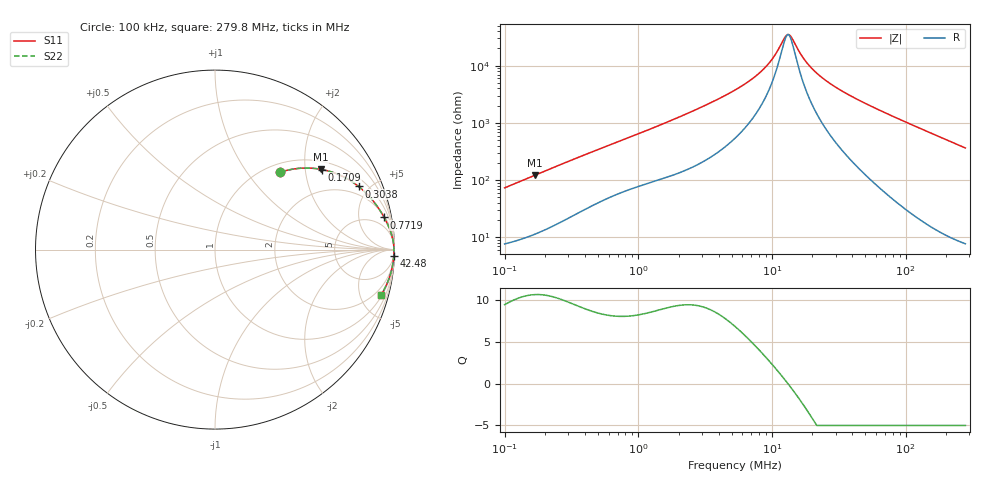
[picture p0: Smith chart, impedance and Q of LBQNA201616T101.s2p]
! LBQNA201616T101  S-PARAMETER MODEL  ( General Type )
! Model Generated by TAIYO YUDEN Corporation (http://www.ty-top.com)
! Version 1.0
! TAIYO YUDEN Control No. 191025NI43SB-FBB
! Copyright(c) 2019 TAIYO YUDEN CO.,LTD. All Rights Reserved.
! Product Description (link to TY-COMPAS)
! https://ds.yuden.co.jp/TYCOMPAS/or/detail?pn=LBQNA201616T101K&u=M
! Products Name : Inductors
! Characteristics :
!  Inductance : 100 uH , SRF(min) : 8.0 MHz , DC Resistance(max) : 5.85 Ohm
!  Rated Current : Saturation :70 mA , Temp Rise : 90 mA (20 degC)
!  Case Size : 2.0 x 1.6 / 0.079 x 0.063 [mm/inch] , Thickness : 1.6 / 0.063 [mm/inch]
!  (Conditions: Temperature = 25 degC , DC Bias Current/Voltage = 0A / 0V)
! External Node Assignments :
!  1  o---GGG---o  2
! GND o---------o GND
! Frequency Range : 0.1MHz  -  279.750408MHz  [ 402 STEP ]
# MHz S RI R 50
! Freq[MHz].  S11 Real  S11 Imag  S21 Real  S21 Imag  S12 Real  S12 Imag  S22 Real  S22 Imag
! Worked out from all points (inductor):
!   401 points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, 100 kHz to 279.8 MHz, reference 50 ohm
!   read as one part in series: L = 116 uH near 104 kHz
!   highest Q = 10.7 at 167.5 kHz (marker M1), where L = 115 uH
!   self-resonance near 13.18 MHz
!   S11 on the Smith chart (normalised r, x): 100 kHz: 1.15, +1.46; 170.9 kHz: 1.23, +2.47; 303.8 kHz: 1.44, +4.30; 771.9 kHz: 2, +10; 42.48 MHz: 5, -53; 279.8 MHz: 1.16, -7.31
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0.1  0.3645 0.4314  0.6355 -0.4314  0.6355 -0.4314  0.3645 0.4314
0.16751  0.5889 0.4475  0.4111 -0.4475  0.4111 -0.4475  0.5889 0.4475
0.170867  0.5974 0.4459  0.4026 -0.4459  0.4026 -0.4459  0.5974 0.4459
0.303772  0.8002 0.3519  0.1998 -0.3519  0.1998 -0.3519  0.8002 0.3519
0.377863  0.8504 0.3061  0.1496 -0.3061  0.1496 -0.3061  0.8504 0.3061
0.771869  0.9424 0.1791  0.0576 -0.1791  0.0576 -0.1791  0.9424 0.1791
1.427803  0.9762 0.1061  0.0238 -0.1061  0.0238 -0.1061  0.9762 0.1061
3.03467  0.9919 0.0506  0.00811 -0.0506  0.00811 -0.0506  0.9919 0.0506
5.289144  0.9955 0.0261  0.0045 -0.0261  0.0045 -0.0261  0.9955 0.0261
7.122612  0.9964 0.0165  0.00364 -0.0165  0.00364 -0.0165  0.9964 0.0165
8.859831  0.9968 0.0103  0.00324 -0.0103  0.00324 -0.0103  0.9968 0.0103
10.38391  0.997 0.0061  0.00304 -0.0061  0.00304 -0.0061  0.997 0.0061
12.41404  0.9971 0.00152  0.00288 -0.00152  0.00288 -0.00152  0.9971 0.00152
13.17541  0.9972 1.32e-05  0.00284 -1.32e-05  0.00284 -1.32e-05  0.9972 1.32e-05
13.98346  0.9972 -0.0015  0.00281 0.0015  0.00281 0.0015  0.9972 -0.0015
16.71734  0.9972 -0.00611  0.00276 0.00611  0.00276 0.00611  0.9972 -0.00611
19.9857  0.9972 -0.0109  0.00277 0.0109  0.00277 0.0109  0.9972 -0.0109
27.45303  0.997 -0.0205  0.003 0.0205  0.003 0.0205  0.997 -0.0205
42.47787  0.9961 -0.0373  0.00395 0.0373  0.00395 0.0373  0.9961 -0.0373
75.51853  0.9922 -0.071  0.00776 0.071  0.00776 0.071  0.9922 -0.071
148.2617  0.9765 -0.1403  0.0235 0.1403  0.0235 0.1403  0.9765 -0.1403
279.7504  0.9258 -0.2517  0.0742 0.2517  0.0742 0.2517  0.9258 -0.2517
